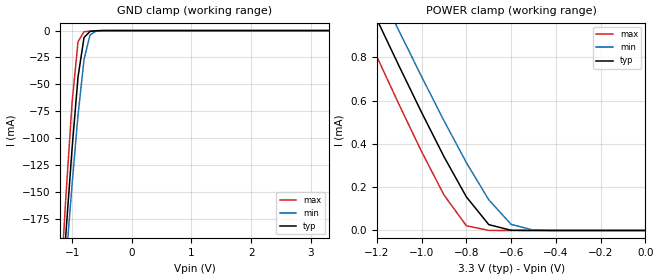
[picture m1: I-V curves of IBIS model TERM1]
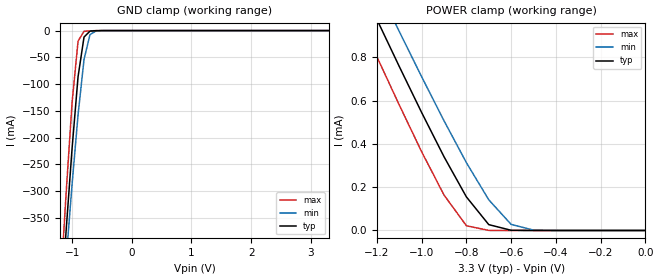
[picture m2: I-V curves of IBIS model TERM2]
|   PERICOM SEMICONDUCTOR CORP
|   IBIS Model of PI4MSD5V9540B
|   Product Family: 4MSD
|   SOIC-8 (W) Package
[IBIS Ver] 3.2
[Comment char] |_char
[File Name] pi4msd5v9540b_w_33v.ibs
[File Rev] 1.0
[Source] File originated at Pericom Semiconductor Corp.
[Date] 09/07/17
[Disclaimer] (C) Copyright PERICOM Semiconductor Corporation
   All rights reserved
  Pericom Semiconductor Corporation hereby grants the user of
  this IBIS model a non-exclusive, nontransferable license to
  use this IBIS model under the following terms.
  This IBIS model is provided on an "AS IS" basis and Pericom
  makes absolutely no warranty with respect to the information
  contained herein. PERICOM DISCLAIMS AND CUSTOMER WAIVES ALL
  WARRANTIES, EXPRESSED OR IMPLIED, INCLUDING WARRANTIES OF
  MERCHANTABILITY OR FITNESS FOR A PARTICULAR PURPOSE. The
  entire risk as to quality and performance is with the customer.
  Accordingly, in no event shall the company be liable for any
  damages, whether in contract or tort, including any lost
  profits or other incidental, consequential, exemplary, or
  punitive damages arising out of the use or application of the
  IBIS model provided in this package. Further, Pericom reserves
  the right to make changes without notice to any product herein
  to improve reliability, function, or design. Pericom does not
  convey any license under patent rights or any other intellectual
  property rights, including those of third parties.
  The user is granted this license only to use the IBIS model
  and is not granted rights to sell, load, rent, lease or license
  the IBIS model in whole or in part, or in modified form to anyone
  other than user. User may modify the IBIS model to suit its specific
  application but rights to derivative works and such modifications
  shall belong to Pericom.
  Pericom is not obligated to provide maintenance or support
  for the licensed IBIS model.
  Contact Pericom at ATTN: APPLICATION ENGINEERING / IBIS MODELS
  2380 Bering Drive, San Jose, CA 95131
[Component] PI4MSD5V9540B
[Manufacturer] Pericom Semiconductor Corp.
[Package]
| variable   typ   min   max
R_pkg   0.05434ohm   0.05079ohm   0.05789ohm
L_pkg   2.52900nH   2.41200nH   2.64600nH
C_pkg   0.17850pF   0.15800pF   0.19900pF
[Pin] signal_name   model_name   R_pin   L_pin   C_pin
1   SCL   TERM2   0.05789   2.64600nH   0.19900pF
2   SDA   TERM2   0.05079   2.41200nH   0.15800pF
3   VCC   POWER   0.05079   2.41200nH   0.15800pF
4   SD0   TERM1   0.05789   2.64600nH   0.19900pF
5   SC0   TERM1   0.05789   2.64600nH   0.19900pF
6   GND   GND   0.05079   2.41200nH   0.15800pF
7   SD1   TERM1   0.05079   2.41200nH   0.15800pF
8   SC1   TERM1   0.05789   2.64600nH   0.19900pF
[Series Switch Groups]
On 1 /
Off 2 /
[Series Pin Mapping]   pin_2   model_name  function_table_group
4   2   SWITCH1   1
5   1   SWITCH1   1
7   2   SWITCH1   2
8   1   SWITCH1   2
|   Model SWITCH1
[Model] SWITCH1
Model_type Series_switch
| variable   typ   min   max
C_comp   6.96pF   6.94pF   6.98pF
[Voltage Range]   3.3000V   3.0000V   3.6000V
[GND Clamp Reference]   0.0000V   0.0000V   0.0000V
[POWER Clamp Reference]   3.3000V   3.0000V   3.6000V
[Temperature Range]   25   85   -40
[On]
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[OFF]
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| Models and submodels in the file (3): SWITCH1 (Series_switch), TERM1 (Terminator), TERM2 (Terminator)
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|   Model TERM1
[Model] TERM1
Model_type Terminator
| variable   typ   min   max
C_comp   2.58pF   2.57pF   2.59pF
[Voltage Range]   3.3000V   3.0000V   3.6000V
[GND Clamp Reference]   0.0000V   0.0000V   0.0000V
[POWER Clamp Reference]   3.3000V   3.0000V   3.6000V
[Temperature Range]   25   85   -40
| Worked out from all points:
|   GND clamp passes 1 mA (typ) near -0.70 V on its own axis
|   POWER clamp passes 1 mA (typ) near -1.21 V on its own axis
[GND Clamp]
| Voltage   I(typ)   I(min)   I(max)
-3.3V     -2.1A      -1.924A    -2.346A
-1.2V     -267.2mA   -286mA     -243.4mA
-1.1V     -186.2mA   -213.2mA   -151.2mA
-1V       -109.4mA   -143.1mA   -66.79mA
-900mV    -42.98mA   -78.43mA   -10.22mA
-800mV    -6.45mA    -26.94mA   -1.105mA
-700mV    -805uA     -4.15mA    -477.3uA
-600mV    -185.9uA   -544.9uA   -115.7uA
3.3V      68.73pA    2.569nA    67.15pA
[POWER Clamp]   |Note: Vtable = Vcc - Voutput
| Voltage   I(typ)   I(min)   I(max)
-3.3V     5.749mA    5.788mA    5.712mA
-1.3V     1.195mA    1.347mA    1.029mA
-1.2V     974.9uA    1.132mA    802.5uA
-1.1V     757.6uA    919.3uA    579.7uA
-1V       544.9uA    710.2uA    363.8uA
-900mV    340.5uA    506.6uA    163.7uA
-800mV    155.1uA    313.2uA    21.83uA
-700mV    27.01uA    141.6uA    235.7nA
-600mV    852.4nA    28.01uA    1.717nA
-500mV    17.67nA    1.596uA    99.08pA
0V        68.73pA    67.71pA    74.93pA
|   Model TERM2
[Model] TERM2
Model_type Terminator
| variable   typ   min   max
C_comp   4.38pF   4.37pF   4.39pF
[Voltage Range]   3.3000V   3.0000V   3.6000V
[GND Clamp Reference]   0.0000V   0.0000V   0.0000V
[POWER Clamp Reference]   3.3000V   3.0000V   3.6000V
[Temperature Range]   25   85   -40
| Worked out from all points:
|   GND clamp passes 1 mA (typ) near -0.70 V on its own axis
|   POWER clamp passes 1 mA (typ) near -1.21 V on its own axis
[GND Clamp]
| Voltage   I(typ)   I(min)   I(max)
-3.3V     -4.214A    -3.861A    -4.708A
-1.2V     -536.3mA   -573.9mA   -488.8mA
-1.1V     -373.8mA   -427.8mA   -304mA
-1V       -219.8mA   -287.2mA   -134.4mA
-900mV    -86.22mA   -157.4mA   -19.74mA
-800mV    -12.06mA   -53.77mA   -1.311mA
-700mV    -1.032mA   -7.522mA   -526.9uA
-600mV    -210.6uA   -734.5uA   -129.9uA
3.3V      125.8pA    2.663nA    123.3pA
[POWER Clamp]   |Note: Vtable = Vcc - Voutput
| Voltage   I(typ)   I(min)   I(max)
-3.3V     5.749mA    5.788mA    5.712mA
-1.3V     1.195mA    1.347mA    1.029mA
-1.2V     974.9uA    1.132mA    802.5uA
-1.1V     757.6uA    919.3uA    579.7uA
-1V       544.9uA    710.2uA    363.8uA
-900mV    340.5uA    506.6uA    163.7uA
-800mV    155.1uA    313.2uA    21.83uA
-700mV    27.01uA    141.6uA    235.8nA
-600mV    852.5nA    28.01uA    1.791nA
-500mV    17.74nA    1.596uA    170.4pA
0V        125.8pA    153.2pA    136.8pA
